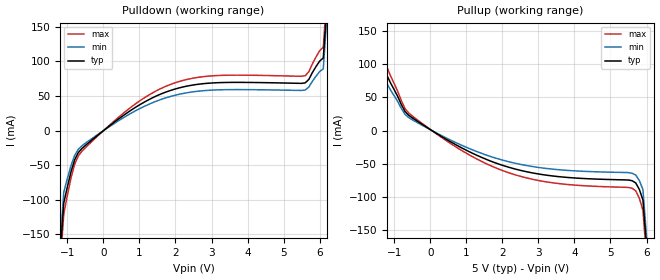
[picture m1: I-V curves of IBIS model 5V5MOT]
[IBIS Ver]   2.1
[File name]   1707_5.ibs
[File Rev]   2.0
[Date]   03/25/2002
[Source]   ICS MicroClock Applications Engineering 2
[Disclaimer] This information is for modeling purposes only, and is
(C) Copyright Integrated Circuit Systems, Inc. 1997-2002
   All rights reserved
ICS hereby grants the user of this IBIS model a non-exclusive,
nontransferable license to use this IBIS model under the following terms.
Before using this IBIS model, the user should read this license.
If the user does not accept these terms,  the IBIS model should be
returned to ICS within 30 days.
   The user is granted this license only to use the IBIS model and
is not granted rights to sell, load, rent, lease or license the IBIS
model in whole or in part, or in modified form to anyone other than
user. User may modify the IBIS model to suit its specific
applications but rights to derivative works and such modifications
shall belong to ICS.
   This IBIS model is provided on an "AS IS" basis and ICS makes
absolutely no warranty with respect to the information contained
herein. ICS DISCLAIMS AND CUSTOMER WAIVES ALL WARRANTIES, EXPRESS
OR IMPLIED, INCLUDING WARRANTIES OF MERCHANTABILITY OR FITNESS FOR
A PARTICULAR PURPOSE. The entire risk as to quality and performance
is with the Customer. ACCORDINGLY, IN NO EVENT SHALL THE COMPANY BE
LIABLE FOR ANY DAMAGES, WHETHER IN CONTRACT OR TORT,INCLUDING ANY
LOST PROFITS OR OTHER INCIDENTAL, CONSEQUENTIAL, EXEMPLARY, OR
PUNITIVE DAMAGES ARISING OUT OF THE USE OR APPLICATION OF THE IBIS
model provided in this package. Further, ICS reserves the right to
make changes without notice to any product herein to improve
reliability, function, or design. ICS does not convey any license
under patent rights or any other intellectual property rights,
including those of third parties.
   ICS is not obligated to provide maintenance or support
for the licensed IBIS model.
[Component]   MK1707
[Manufacturer] Integrated Circuit Systems Inc.
[Package]
|   typ   min   max
R_pkg   40m   35m   45m
L_pkg   1.65nH   1.35nH   1.95nH
C_pkg   0.24pF   0.14pF   0.34pF
[pin]   signal_name   model_name   R_pin   L_pin   C_pin
   4   CLK   5V5MOT
| Models and submodels in the file (1): 5V5MOT (Output)
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|   MK1707 5V Clock Drive Model
| This model is suitable for all single output pins on the
| MK1707
[Model]   5V5MOT
Model_type   Output
Polarity   Non-Inverting
|   typ   min   max
C_comp   5pF   4pF   6pF
|   typ   min   max
[Voltage range]  5.0V   4.5V   5.5V
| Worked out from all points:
|   slope of the pulldown table from 0 to 0.75 V, typ, clamps not added: 25.8 ohm
|   slope of the pullup table from 0 to 0.75 V, typ, clamps not added: 31.1 ohm
[pulldown]
|Voltage I (typ)   I (min)   I (max)
-5V       -3A        -3A        -3A
-1.1V     -105mA     -89.25mA   -120.8mA
-900mV    -59.85mA   -50.87mA   -68.83mA
-800mV    -42.79mA   -36.37mA   -49.21mA
-600mV    -26.26mA   -22.32mA   -30.2mA
800mV     30.54mA    25.96mA    35.12mA
1.8V      56.89mA    48.35mA    65.42mA
3V        68.74mA    58.43mA    79.05mA
5.6V      68.97mA    58.63mA    79.32mA
6V        100.4mA    85.38mA    115.5mA
6.1V      105mA      89.25mA    120.7mA
10V       3A         3A         3A
[pullup]
|Voltage I (typ)   I (min)   I (max)
-5V       3A         3A         3A
-1.2V     83.12mA    70.65mA    95.59mA
-700mV    28.74mA    24.42mA    33.04mA
-600mV    23.15mA    19.68mA    26.63mA
800mV     -24.16mA   -20.54mA   -27.79mA
1.9V      -50.71mA   -43.1mA    -58.32mA
3.3V      -68.09mA   -57.87mA   -78.3mA
5.6V      -75.91mA   -64.52mA   -87.3mA
5.7V      -79.25mA   -67.36mA   -91.14mA
5.8V      -89.07mA   -75.71mA   -102.4mA
5.9V      -105mA     -89.25mA   -120.7mA
10V       -3A        -3A        -3A
[Ramp]
|   typ   min   max
dV/dt_r   1.70/1.12n   1.62/1.23n   1.79/1.02n
dV/dt_f   1.93/0.85n   1.83/0.94n   2.03/0.77n
